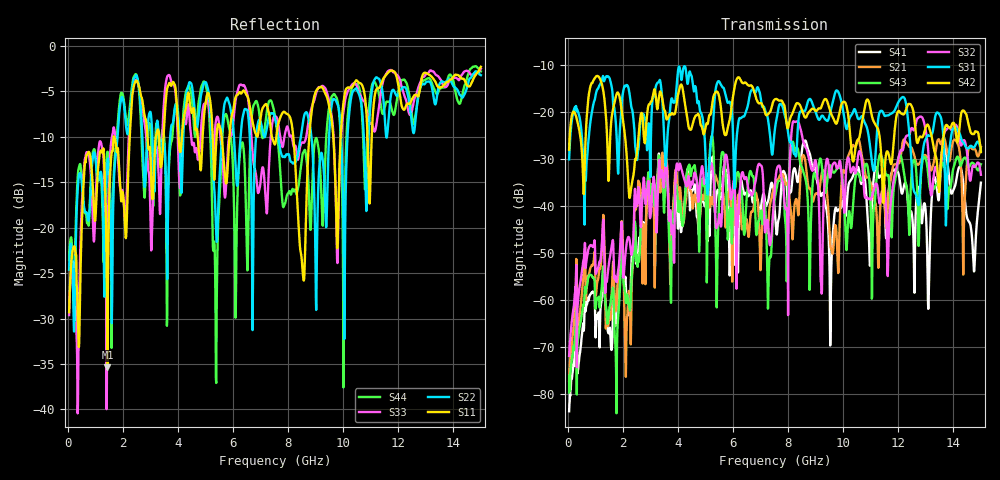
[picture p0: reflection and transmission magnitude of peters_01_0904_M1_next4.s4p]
# MHZ S RI R 50.00
! FREQ  S11  S12  S13  S14
!  S21  S22  S23  S24
!  S31  S32  S33  S34
!  S41  S42  S43  S44
!  REAL  IMAG  REAL  IMAG  REAL  IMAG  REAL  IMAG
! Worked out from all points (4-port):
!   1496 points, 50 MHz to 15 GHz, reference 50 ohm
!   strongest paths, dB at 50 MHz, 3.79 GHz, 7.53 GHz, 11.27 GHz, 15 GHz:
!     S42: -28.0, -20.3, -17.3, -23.7, -28.5
!     S31: -30.1, -17.2, -23.3, -21.6, -28.2
!     S32: -71.8, -45.8, -35.0, -37.0, -33.4
!     S43: -79.6, -45.7, -38.0, -30.9, -31.1
!     S21: -77.2, -44.7, -35.3, -52.4, -27.5
!     S41: -83.6, -42.2, -42.4, -33.5, -35.0
!   lowest |S11| = -35.3 dB at 1.44 GHz (marker M1), VSWR 1.03, Z = 49.2 - j1.52 ohm
!   |S11| at or under -10 dB: start of sweep to 1.667 GHz; 1.686 GHz to 2.251 GHz (565.6 MHz wide, 28.7 % of centre); 8.189 GHz to 8.769 GHz (579.5 MHz wide, 6.83 % of centre)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
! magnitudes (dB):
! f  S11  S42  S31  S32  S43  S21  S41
! 50 MHz  -29.3  -28.0  -30.1  -71.8  -79.6  -77.2  -83.6
! 1.44 GHz  -35.3  -27.1  -12.5  -55.0  -65.0  -65.4  -65.9
! 3.36 GHz  -13.0  -15.7  -13.5  -33.5  -33.3  -37.1  -34.7
! 7.31 GHz  -7.5  -20.3  -23.3  -46.9  -52.3  -41.5  -37.8
! 8.17 GHz  -9.4  -20.2  -27.5  -22.3  -26.3  -47.0  -33.3
! 9.2 GHz  -4.5  -19.1  -21.0  -56.2  -30.4  -33.7  -37.9
! 15 GHz  -2.3  -28.5  -28.2  -33.4  -31.1  -27.5  -35.0
